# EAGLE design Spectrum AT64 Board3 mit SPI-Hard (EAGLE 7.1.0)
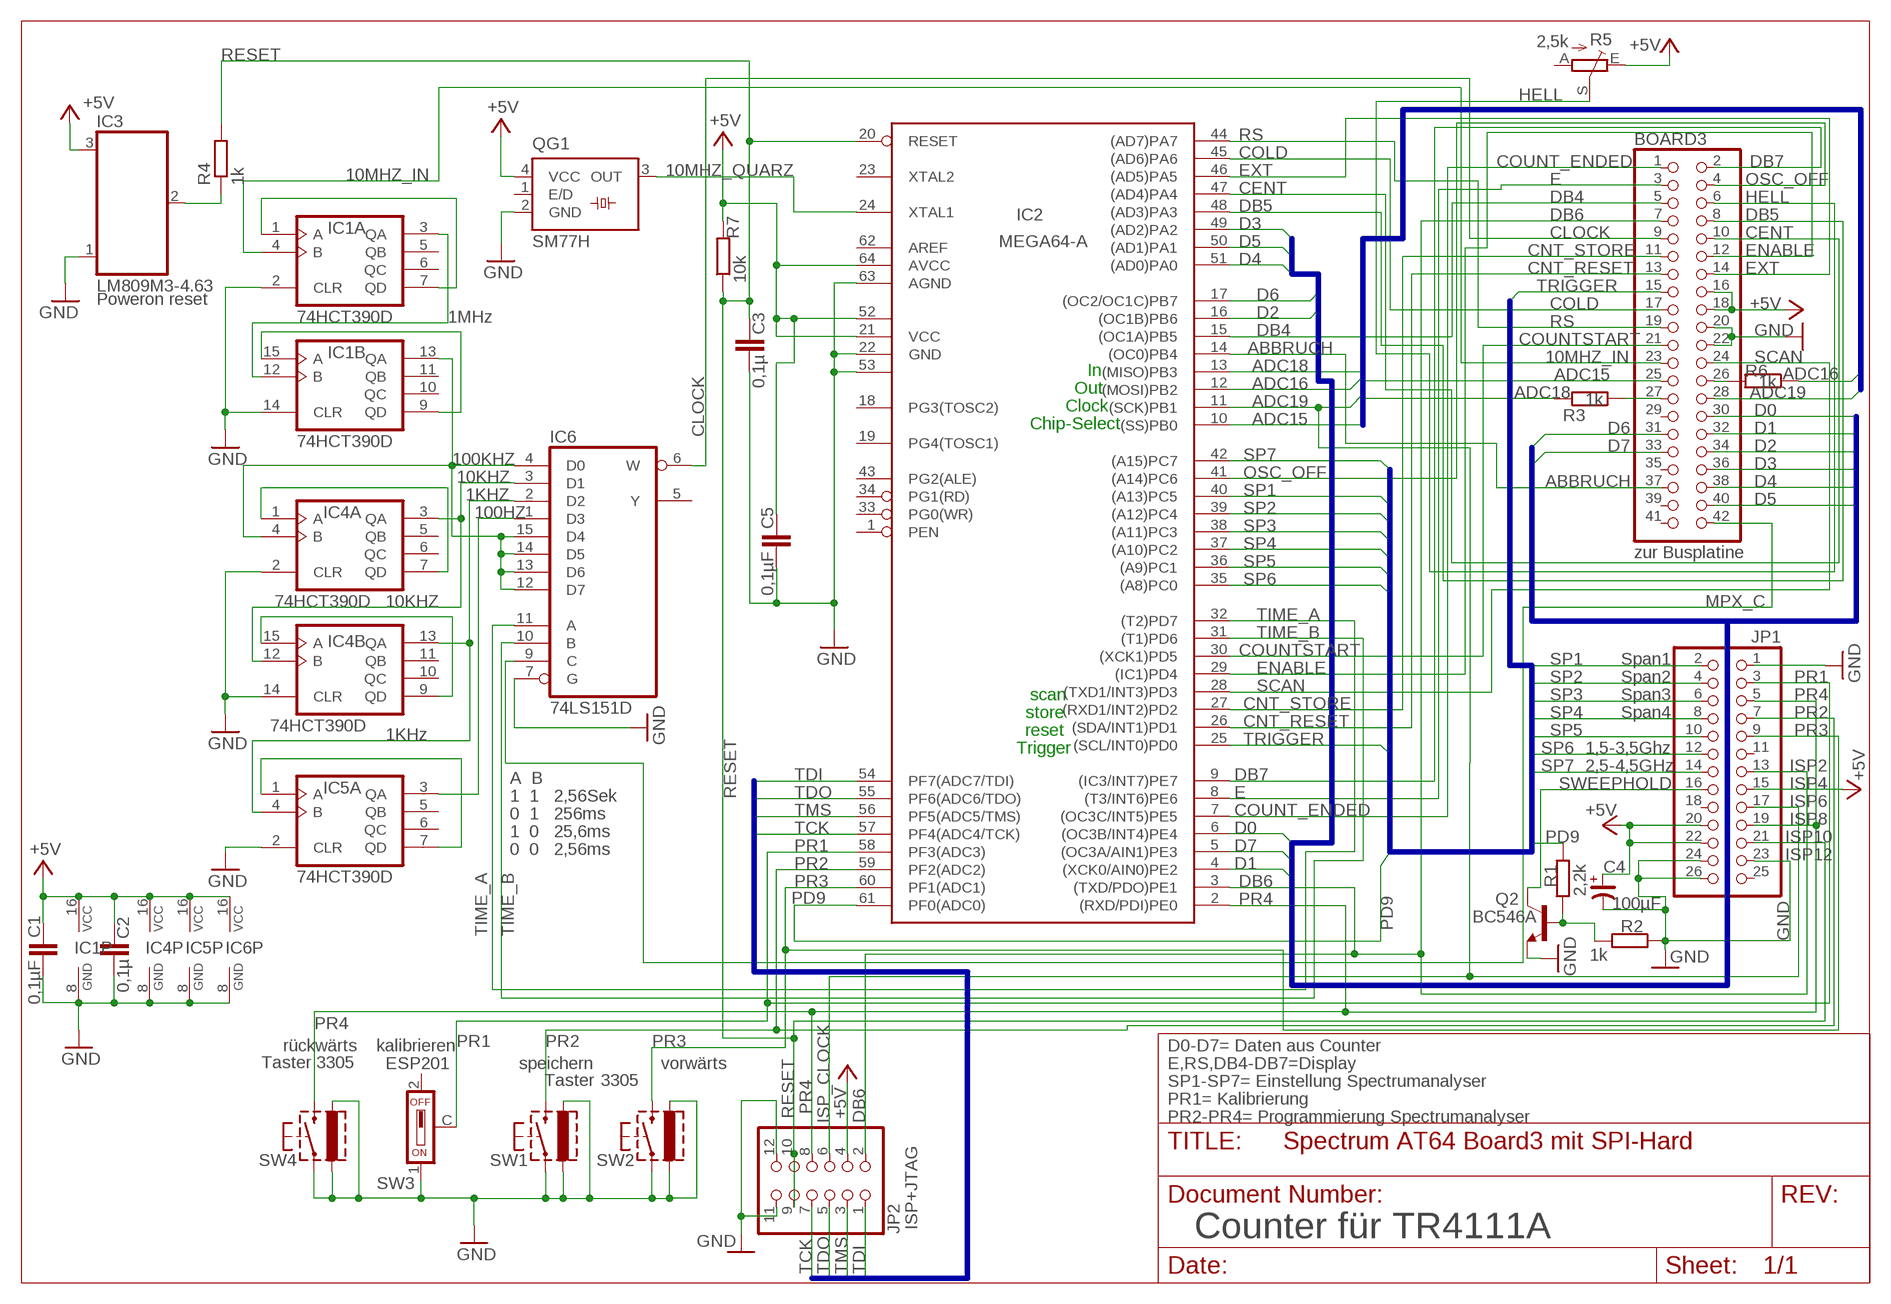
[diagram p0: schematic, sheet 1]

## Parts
BOARD3  zur Busplatine  PINHD-2X21_2.54-90°  [2X21/90]
C1  0,1µF  C-EUC0805  [C0805]
C2  0,1µ  C-EU025-025X050  [C025-025X050]
C3  0,1µ  C-EUC0805K  [C0805K]
C4  100µF  CP_SV-D  [CSV-D]
C5  0,1µF  C-EUC0805  [C0805]
IC1  74HCT390D  [SO16]
IC2  MEGA64-A  [TQFP64]
IC3  LM809M3-4.63  [SOT23]
IC4  74HCT390D  [SO16]
IC5  74HCT390D  [SO16]
IC6  74LS151D  74S151D  [SO16]
JP1  PINHD-2X13_2.54-90°  [2X13/90]
JP2  ISP+JTAG  PINHD-2X06_2.54-90°  [2X06/90]
Q2  BC546A  [TO92-EBC]
QG1  SM77H  [SM77H]
R1  2,2k  R-EU_R0805  [R0805]
R2  1k  R-EU_R0805  [R0805]
R3  1k  R-EU_R0805  [R0805]
R4  1k  R-EU_R0805  [R0805]
R5  2,5k  TRIM_EU-CA6H  [CA6H]
R6  1k  R-EU_R0805  [R0805]
R7  10k  WIDERSTAND_10  [207.10]
SW1  Taster  SW-PUSH-90  [SW-PUSH-90]
SW2  3305  SW-PUSH-90  [SW-PUSH-90]
SW3  ESP201  [ESP201]
SW4  Taster 3305  SW-PUSH-90  [SW-PUSH-90]

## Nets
1KHZ: IC4.13(B:QA) IC5.4(A:B) IC6.2(D2)
1MHZ: IC1.3(A:QA) IC1.12(B:B)
10KHZ: IC4.3(A:QA) IC4.12(B:B) IC6.3(D1)
10MHZ_IN: BOARD3.23 IC1.4(A:B)
10MHZ_QUARZ: IC2.24(XTAL1) QG1.3(OUT)
100HZ: IC5.3(A:QA) IC6.1(D3)
100KHZ: IC1.13(B:QA) IC4.4(A:B) IC6.4(D0) IC6.12(D7) IC6.13(D6) IC6.14(D5) IC6.15(D4)
+5V: BOARD3.16 BOARD3.18 C1.2 C2.1 C4.+ C5.2 IC1.16(P:VCC) IC2.21(VCC) IC2.52(VCC1) IC2.64(AVCC) IC3.3(VCC) IC4.16(P:VCC) IC5.16(P:VCC) IC6.16(VCC) JP1.15 JP1.20 JP1.22 JP2.4 QG1.4(VCC) R5.E R7.2
ABBRUCH: BOARD3.37 IC2.14((OC0)PB4)
ADC15: BOARD3.25 IC2.10((SS)PB0)
ADC16: IC2.12((MOSI)PB2) R6.1
ADC18: IC2.13((MISO)PB3) R3.2
ADC19: BOARD3.28 IC2.11((SCK)PB1) JP1.17 JP2.6
CENT: BOARD3.10 IC2.47((AD4)PA4)
CLOCK: BOARD3.9 IC6.6(W)
CNT_RESET: BOARD3.13 IC2.26((SDA/INT1)PD1)
CNT_STORE: BOARD3.11 IC2.27((RXD1/INT2)PD2)
COLD: BOARD3.17 IC2.45((AD6)PA6)
COUNT_ENDED: BOARD3.1 IC2.7((OC3C/INT5)PE5)
COUNTSTART: BOARD3.21 IC2.30((XCK1)PD5)
D0: BOARD3.30 IC2.6((OC3B/INT4)PE4)
D1: BOARD3.32 IC2.4((XCK0/AIN0)PE2)
D2: BOARD3.34 IC2.16((OC1B)PB6)
D3: BOARD3.36 IC2.49((AD2)PA2)
D4: BOARD3.38 IC2.51((AD0)PA0)
D5: BOARD3.40 IC2.50((AD1)PA1)
D6: BOARD3.31 IC2.17((OC2/OC1C)PB7)
D7: BOARD3.33 IC2.5((OC3A/AIN1)PE3)
DB4: BOARD3.5 IC2.15((OC1A)PB5)
DB5: BOARD3.8 IC2.48((AD3)PA3)
DB6: BOARD3.7 IC2.3((TXD/PDO)PE1) JP1.13 JP2.2
DB7: BOARD3.2 IC2.9((IC3/INT7)PE7)
E: BOARD3.3 IC2.8((T3/INT6)PE6)
ENABLE: BOARD3.12 IC2.29((IC1)PD4)
EXT: BOARD3.14 IC2.46((AD5)PA5)
GND: BOARD3.20 BOARD3.22 C1.1 C2.2 C3.2 C4.- C5.1 IC1.2(A:CLR) IC1.8(P:GND) IC1.14(B:CLR) IC2.22(GND) IC2.53(GND1) IC2.63(AGND) IC3.1(GND) IC4.2(A:CLR) IC4.8(P:GND) IC4.14(B:CLR) IC5.2(A:CLR) IC5.8(P:GND) IC6.7(G) IC6.8(GND) JP1.1 JP1.23 JP1.24 JP1.26 JP2.11 JP2.12 Q2.E QG1.2(GND) R2.1 SW1.1 SW1.3(G1) SW1.4(G2) SW2.1 SW2.3(G1) SW2.4(G2) SW3.1 SW4.1 SW4.3(G1) SW4.4(G2)
HELL: BOARD3.6 R5.S
MPX_C: BOARD3.42 IC6.9(C)
N$2: IC3.2(/RESET) R4.1
N$4: IC1.1(A:A) IC1.7(A:QD)
N$5: BOARD3.27 R3.1
N$6: Q2.B R1.1 R2.2
N$7: BOARD3.26 R6.2
N$11: IC1.9(B:QD) IC1.15(B:A)
N$15: IC5.1(A:A) IC5.7(A:QD)
N$17: IC4.1(A:A) IC4.7(A:QD)
N$18: IC4.9(B:QD) IC4.15(B:A)
OSC_OFF: BOARD3.4 IC2.41((A14)PC6)
PD9: IC2.61(PF0(ADC0)) R1.2
PR1: IC2.58(PF3(ADC3)) JP1.3 SW3.C
PR2: IC2.59(PF2(ADC2)) JP1.7 SW1.2(S1)
PR3: IC2.60(PF1(ADC1)) JP1.9 SW2.2(S1)
PR4: IC2.2((RXD/PDI)PE0) JP1.5 JP1.19 JP2.8 SW4.2(S1)
RESET: C3.1 IC2.20(RESET) JP1.21 JP2.9 JP2.10 R4.2 R7.1
RS: BOARD3.19 IC2.44((AD7)PA7)
SCAN: BOARD3.24 IC2.28((TXD1/INT3)PD3)
SP1: IC2.40((A13)PC5) JP1.2
SP2: IC2.39((A12)PC4) JP1.4
SP3: IC2.38((A11)PC3) JP1.6
SP4: IC2.37((A10)PC2) JP1.8
SP5: IC2.36((A9)PC1) JP1.10
SP6: IC2.35((A8)PC0) JP1.12
SP7: IC2.42((A15)PC7) JP1.14
SWEEPHOLD: JP1.16 Q2.C
TCK: IC2.57(PF4(ADC4/TCK)) JP2.7
TDI: IC2.54(PF7(ADC7/TDI)) JP2.1
TDO: IC2.55(PF6(ADC6/TDO)) JP2.5
TIME_A: IC2.32((T2)PD7) IC6.11(A)
TIME_B: IC2.31((T1)PD6) IC6.10(B)
TMS: IC2.56(PF5(ADC5/TMS)) JP2.3
TRIGGER: BOARD3.15 IC2.25((SCL/INT0)PD0)
Unconnected: BOARD3.29 BOARD3.35 BOARD3.39 BOARD3.41 IC1.5(A:QB) IC1.6(A:QC) IC1.10(B:QC) IC1.11(B:QB) IC2.1(PEN) IC2.18(PG3(TOSC2)) IC2.19(PG4(TOSC1)) IC2.23(XTAL2) IC2.33(PG0(WR)) IC2.34(PG1(RD)) IC2.43(PG2(ALE)) IC2.62(AREF) IC4.5(A:QB) IC4.6(A:QC) IC4.10(B:QC) IC4.11(B:QB) IC5.5(A:QB) IC5.6(A:QC) IC5.9(B:QD) IC5.10(B:QC) IC5.11(B:QB) IC5.12(B:B) IC5.13(B:QA) IC5.14(B:CLR) IC5.15(B:A) IC6.5(Y) JP1.11 JP1.18 JP1.25 QG1.1(E/D) R5.A SW3.2

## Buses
ADC[15..19]
D[0..7]
SP[1..10],TRIGGER,PD9
TDI,TDO,TMS,TCK,RESET

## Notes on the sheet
- Poweron reset
- 1MHz
- In
- Out
- Clock
- Chip-Select
- 10KHZ
- Span1
- Span2
- scan | Span3
- store | Span4
- 1KHz | reset
- Trigger | 1,5-3,5Ghz
- A  B | 2,5-4,5GHz | ISP2
- 1  1   2,56Sek | ISP4
- 0  1   256ms | ISP6
- 1  0   25,6ms | ISP8
- 0  0   2,56ms | ISP10
- ISP12
- rückwärts | kalibrieren | D0-D7= Daten aus Counter
- speichern | vorwärts | E,RS,DB4-DB7=Display
- SP1-SP7= Einstellung Spectrumanalyser
- PR1= Kalibrierung
- ISP_CLOCK | PR2-PR4= Programmierung Spectrumanalyser
- Counter für TR4111A

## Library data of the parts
BOARD3 = pinhead-2:PINHD-2X21: PIN HEADER
C1-C3 C5 = rcl:C-EU: CAPACITOR, European symbol
C4 = rc-master-smd:CP_: POLARIZED CAP
IC1 IC4 IC5 = 74xx-eu:74*390: Dual 4-bit decade and binary COUNTER
IC2 = atmel:MEGA64: MICROCONTROLLER 64 Kbytes FLASH 4 Kbytes SRAM 2 Kbytes EEPROM DUAL USART 8-channel 10 bit ADC Source: avr.lbr
IC3 = 1Eigene:LM809M3-4.63
IC6 = 74xx-eu:74*151: Data SELECTOR/MULTIPLEXER
JP1 = pinhead-2:PINHD-2X13: PIN HEADER
JP2 = pinhead-2:PINHD-2X06: PIN HEADER
Q2 = transistor-npn:BC546*: NPN Transistor
QG1 = crystal:SM77H: 3.3V CMOS Clock Oscillator Source: www.pletronics.com .. sm77h%203.3v.pdf
R1-R4 R6 = rcl:R-EU_: RESISTOR, European symbol
R5 = pot:TRIM_EU-: POTENTIOMETER
R7 = 1Eigene:WIDERSTAND_10
SW1 SW2 SW4 = 1Eigene:SW-PUSH-90
SW3 = 1Eigene:ESP201

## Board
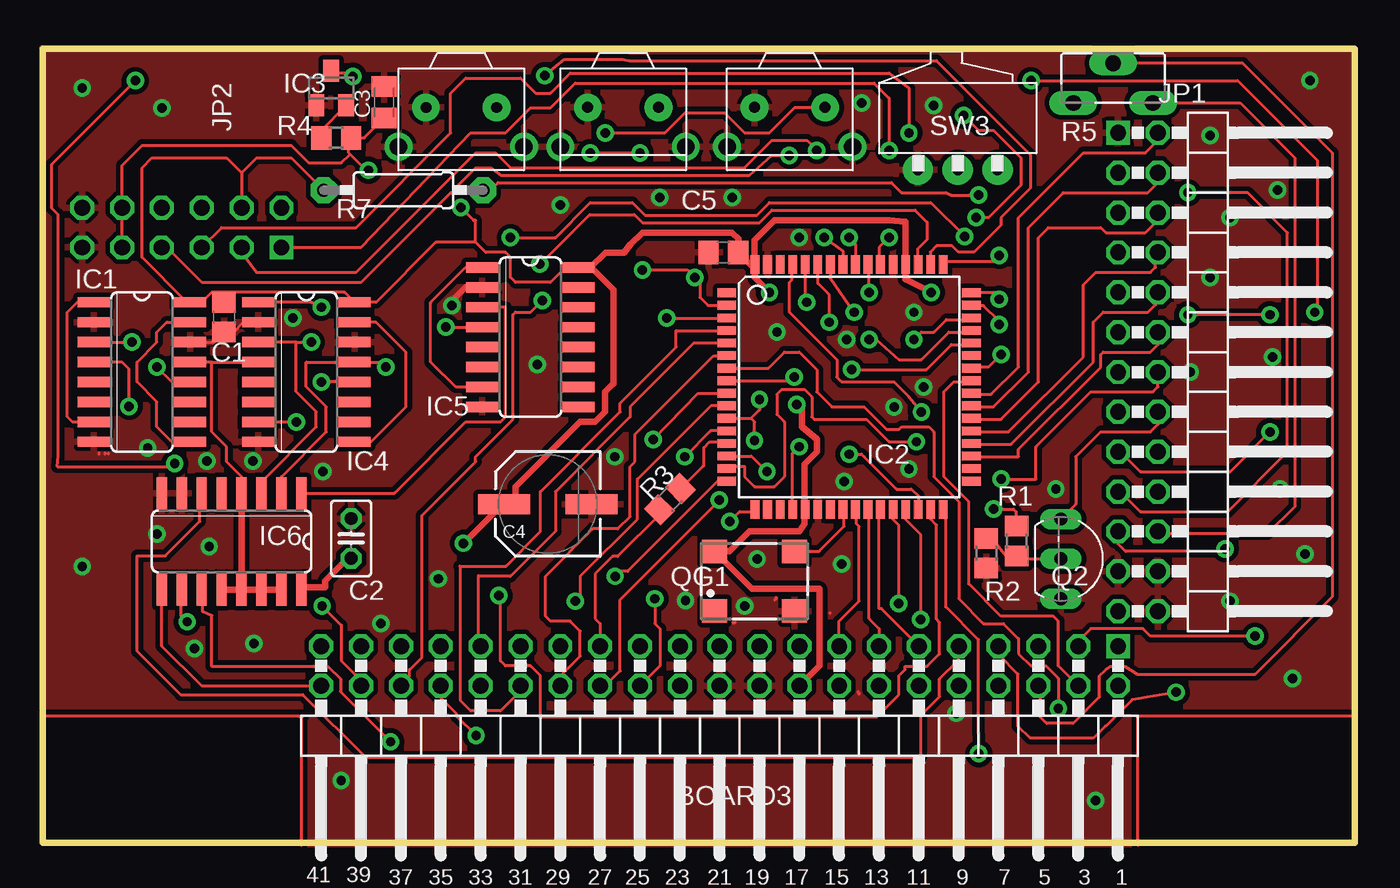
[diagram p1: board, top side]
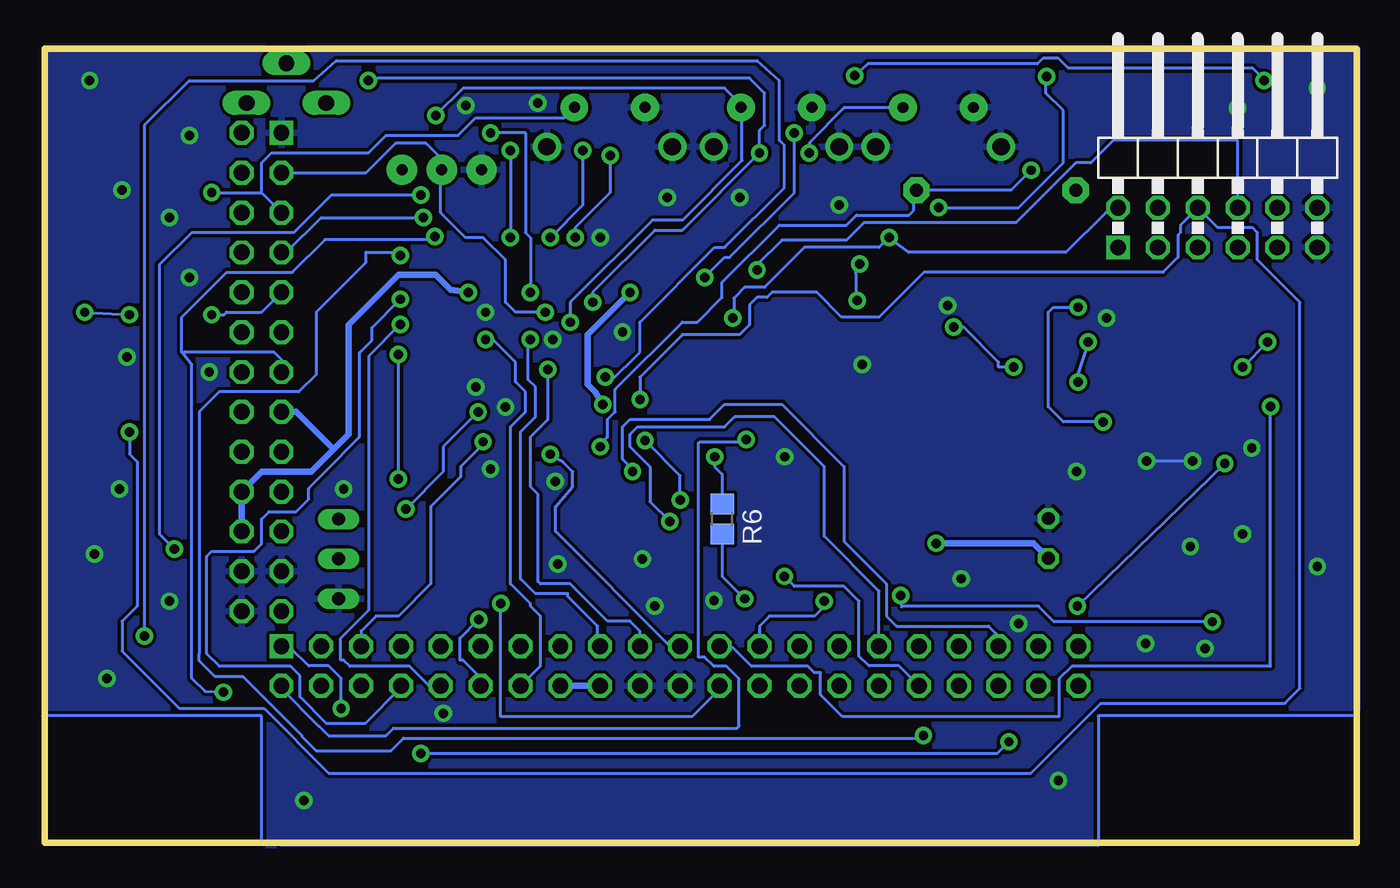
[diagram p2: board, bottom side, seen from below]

Size 83.63 x 50.58 mm. Coordinates in mm from the lower left corner, seen from the top.
Outline: 0,0 83.63,0 83.63,50.58 0,50.58 0,0
Copper layers (1*16): Top 0.035mm / dielectric 1.5mm / Bottom 0.035mm
Design rules "default *": minimum track width 0.2mm, minimum drill 0.6mm, track to track 0.2mm, track to pad 0.2mm, pad to pad 0.2mm, via to via 0.2mm, smd to smd 0.2mm, copper to edge 0mil, drill to drill 0.4mm, minimum pad ring 10mil, minimum via ring 10mil, stop-mask expansion 4mil, vias tented up to drill 0mil, thermal gap 10mil

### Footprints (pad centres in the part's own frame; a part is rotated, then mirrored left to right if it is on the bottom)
2X21/90 = drill 1.016 square: 1 -24.13,-6.35 | drill 1.016 octagon: 2 -24.13,-3.81; 3 -21.59,-6.35; 4 -21.59,-3.81; 5 -19.05,-6.35; 6 -19.05,-3.81; 7 -16.51,-6.35; 8 -16.51,-3.81; 9 -13.97,-6.35; 10 -13.97,-3.81; 11 -11.43,-6.35; 12 -11.43,-3.81; 13 -8.89,-6.35; 14 -8.89,-3.81; 15 -6.35,-6.35; 16 -6.35,-3.81; 17 -3.81,-6.35; 18 -3.81,-3.81; 19 -1.27,-6.35; 20 -1.27,-3.81; 21 1.27,-6.35; 22 1.27,-3.81; 23 3.81,-6.35; 24 3.81,-3.81; 25 6.35,-6.35; 26 6.35,-3.81; 27 8.89,-6.35; 28 8.89,-3.81; 29 11.43,-6.35; 30 11.43,-3.81; 31 13.97,-6.35; 32 13.97,-3.81; 33 16.51,-6.35; 34 16.51,-3.81; 35 19.05,-6.35; 36 19.05,-3.81; 37 21.59,-6.35; 38 21.59,-3.81; 39 24.13,-6.35; 40 24.13,-3.81; 41 26.67,-6.35; 42 26.67,-3.81
C0805 = smd 1.3 x 1.5: 1 -0.95,0; 2 0.95,0
C025-025X050 = drill 0.813 octagon: 1 -1.27,0; 2 1.27,0
C0805K = smd 1.3 x 1.6: 1 -1,0; 2 1,0
CSV-D = smd 3.302 x 1.27: + -2.794,0; - 2.794,0
SO16 = smd 0.66 x 2.032: 1 -4.445,-3.073; 2 -3.175,-3.073; 3 -1.905,-3.073; 4 -0.635,-3.073; 5 0.635,-3.073; 6 1.905,-3.073; 7 3.175,-3.073; 8 4.445,-3.073; 9 4.445,3.073; 10 3.175,3.073; 11 1.905,3.073; 12 0.635,3.073; 13 -0.635,3.073; 14 -1.905,3.073; 15 -3.175,3.073; 16 -4.445,3.073
TQFP64 = smd 1.194 x 0.559: 1 -7.8,6; 2 -7.8,5.2; 3 -7.8,4.4; 4 -7.8,3.6; 5 -7.8,2.8; 6 -7.8,2; 7 -7.8,1.2; 8 -7.8,0.4; 9 -7.8,-0.4; 10 -7.8,-1.2; 11 -7.8,-2; 12 -7.8,-2.8; 13 -7.8,-3.6; 14 -7.8,-4.4; 15 -7.8,-5.2; 16 -7.8,-6; 33 7.8,-6; 34 7.8,-5.2; 35 7.8,-4.4; 36 7.8,-3.6; 37 7.8,-2.8; 38 7.8,-2; 39 7.8,-1.2; 40 7.8,-0.4; 41 7.8,0.4; 42 7.8,1.2; 43 7.8,2; 44 7.8,2.8; 45 7.8,3.6; 46 7.8,4.4; 47 7.8,5.2; 48 7.8,6 | smd 0.559 x 1.194: 17 -6,-7.8; 18 -5.2,-7.8; 19 -4.4,-7.8; 20 -3.6,-7.8; 21 -2.8,-7.8; 22 -2,-7.8; 23 -1.2,-7.8; 24 -0.4,-7.8; 25 0.4,-7.8; 26 1.2,-7.8; 27 2,-7.8; 28 2.8,-7.8; 29 3.6,-7.8; 30 4.4,-7.8; 31 5.2,-7.8; 32 6,-7.8; 49 6,7.8; 50 5.2,7.8; 51 4.4,7.8; 52 3.6,7.8; 53 2.8,7.8; 54 2,7.8; 55 1.2,7.8; 56 0.4,7.8; 57 -0.4,7.8; 58 -1.2,7.8; 59 -2,7.8; 60 -2.8,7.8; 61 -3.6,7.8; 62 -4.4,7.8; 63 -5.2,7.8; 64 -6,7.8
SOT23 = smd 1 x 1.4: 1 -0.95,-1.1; 2 0.95,-1.1; 3 0,1.1
2X13/90 = drill 1.016 square: 1 -15.24,-6.35 | drill 1.016 octagon: 2 -15.24,-3.81; 3 -12.7,-6.35; 4 -12.7,-3.81; 5 -10.16,-6.35; 6 -10.16,-3.81; 7 -7.62,-6.35; 8 -7.62,-3.81; 9 -5.08,-6.35; 10 -5.08,-3.81; 11 -2.54,-6.35; 12 -2.54,-3.81; 13 0,-6.35; 14 0,-3.81; 15 2.54,-6.35; 16 2.54,-3.81; 17 5.08,-6.35; 18 5.08,-3.81; 19 7.62,-6.35; 20 7.62,-3.81; 21 10.16,-6.35; 22 10.16,-3.81; 23 12.7,-6.35; 24 12.7,-3.81; 25 15.24,-6.35; 26 15.24,-3.81
2X06/90 = drill 1.016 square: 1 -6.35,-6.35 | drill 1.016 octagon: 2 -6.35,-3.81; 3 -3.81,-6.35; 4 -3.81,-3.81; 5 -1.27,-6.35; 6 -1.27,-3.81; 7 1.27,-6.35; 8 1.27,-3.81; 9 3.81,-6.35; 10 3.81,-3.81; 11 6.35,-6.35; 12 6.35,-3.81
TO92-EBC = drill 0.813 long: B 0,-1.27; C -2.54,-1.27; E 2.54,-1.27
SM77H = smd 1.6 x 1.5: 1 -2.55,-1.9; 2 2.55,-1.9; 3 2.55,1.9; 4 -2.55,1.9
R0805 = smd 1.3 x 1.5: 1 -0.95,0; 2 0.95,0
CA6H = drill 1.016 long: A -2.54,0; E 2.54,0; S 0,2.54
207.10 = drill 0.813 pad 1.676 octagon: 1 -5.08,0; 2 5.08,0
SW-PUSH-90 = drill 0.7 pad 1.778: 1 1.75,4; 2 6.25,4 | drill 1.1 pad 1.778: 3 0,1.5; 4 8,1.5
ESP201 = drill 0.7 pad 1.93: 1 -2.54,-2.54; 2 2.54,-2.54; C 0,-2.54

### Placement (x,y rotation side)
BOARD3  44.42,6.17 180 top
C1  11.56,33.48 90 top
C2  19.66,19.38 90 top
C3  21.77,47.18 90 top
C4  32.2,21.57 0 top
C5  43.39,37.6 0 top
IC1  6.32,29.98 270 top
IC2  51.41,29.03 0 top
IC3  18.39,48.08 0 top
IC4  16.8,29.98 270 top
IC5  31.09,32.21 270 top
IC6  12.04,19.19 180 top
JP1  74.9,29.98 270 top
JP2  8.86,44.27 0 bottom
Q2  66.17,18.08 270 top
QG1  45.38,16.65 0 top
R1  62.09,19.21 90 top
R2  60.15,18.44 90 top
R3  39.98,21.89 45 top
R4  18.71,44.91 0 top
R5  68.24,47.13 0 top
R6  40.46,20.62 270 bottom
R7  22.99,41.57 180 top
SW1  32.99,42.84 0 top
SW2  22.68,42.84 0 top
SW3  58.33,45.42 0 top
SW4  43.63,42.84 0 top

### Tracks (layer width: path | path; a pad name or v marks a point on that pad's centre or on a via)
1KHZ  (via drill 0.6 pad 0.7)
  Top 0.2: IC6.2 15.21,23.32 18.07,26.17 18.07,27.76 16.8,29.03 16.8,30.62 IC4.13 21.56,30.62 v21.88,30.3 | v25.69,32.84 IC5.4
  Bottom 0.2: v21.88,30.3 22.83,30.3 22.83,30.62 25.06,32.84 v25.69,32.84
1MHZ  (via drill 0.6 pad 0.7)
  Top 0.2: IC1.12 9.5,29.4 8.18,29.4 v7.28,30.3 | IC1.3 v5.69,31.89
  Bottom 0.2: v5.69,31.89 v7.28,30.3
10KHZ  (via drill 0.6 pad 0.7)
  Top 0.2: IC4.12 19.95,29.4 17.8,29.4 v17.75,29.35 | IC6.3 13.94,23 17.44,26.49 17.44,27.44 16.17,28.71 16.17,31.89 | 16.17,31.89 IC4.3 | 16.17,31.89 v17.12,31.89
  Bottom 0.2: v17.75,29.35 17.75,29.99 v17.12,31.89
10MHZ_IN  (via drill 0.6 pad 0.7)
  Top 0.2: v5.5,27.8 5.5,30.17 5.05,30.62 IC1.4
  Bottom 0.2: v5.5,27.8 5.5,11.22 18.17,11.22 18.97,10.42 18.97,8.02 32.77,8.02 34.17,9.42 34.17,10.82 34.57,10.82 34.97,11.22 38.57,11.22 39.77,12.42 40.57,12.42 BOARD3.23
10MHZ_QUARZ
  Top 0.2: QG1.3 49.5,18.55 51.09,20.14 51.09,21.15 IC2.24
100HZ
  Top 0.2: IC6.1 16.61,22.27 22.42,22.27 26.96,26.81 29.18,26.81 29.5,27.13 29.5,34.11 IC5.3
100KHZ
  Top 0.2: IC6.4 12.67,23.32 11.72,24.27 11.72,25.22 10.77,26.17 10.77,30.62 | 10.77,30.62 IC1.13 | 10.77,30.62 IC4.4
  Top 0.406: IC6.15 IC6.14 IC6.13 | IC6.12 IC6.13 | IC6.13 IC6.4
+5V  (via drill 0.6 pad 0.7)
  Top 0.2: 45.11,36.83 IC2.64 45.38,36.86 | IC2.21 48.55,21.17 | 48.55,21.29 IC2.21 | IC2.21 48.55,21.13 | 49.5,11.41 49.5,11.25 | IC6.16 16.61,16.27 | 19.61,18.27 C2.1 | 30.97,21.62 30.14,21.62 29.57,21.62 C4.+ 29.37,21.62 | IC4.16 19.75,34.6 | v19.77,48.82 19.77,49.02 18.57,49.02 IC3.3 | IC4.16 19.95,34.6 | 34.97,36.62 34.9,36.62 34.17,36.62 IC5.16 33.97,36.82 33.48,36.82 32.36,35.7 30.14,35.7 29.82,36.02 29.82,37.29 29.5,37.6 28.23,37.6 27.6,38.24 | 36.36,29.22 36.37,29.22 | R7.2 15.85,43.64 13.63,43.64 12.67,42.68 | 12.67,42.68 JP2.4 | 11.56,35.06 19.24,35.06 IC4.16 | 11.56,35.06 10.77,35.06 10.13,34.43 IC1.16 9.18,34.43 6.32,37.29 6.32,43 6.96,43.64 11.72,43.64 12.67,42.68 | 27.6,38.24 27.6,39.64 27.46,39.64 v26.64,40.46 | 27.6,38.24 25.06,38.24 21.25,34.43 IC4.16 | R5.E 76.33,47.13 79.83,43.64 79.83,21.41 78.08,19.67 71.25,19.67 JP1.22 | C1.2 11.56,35.06
  Top 0.406: 45.11,36.83 C5.2 44.34,38.48 43.95,38.88 38.23,38.88 37.48,38.12 37.06,37.59 35.86,37.59 34.9,36.62 | IC2.64 45.41,35.99 v46.33,35.06 | 45.38,36.86 45.38,38.4 46.65,39.67 53.95,39.67 55.01,39.56 IC2.52 55.01,35.91 v56.65,35.06 | 49.5,11.41 49.5,14.27 49.5,16.17 45.2,16.17 QG1.4 43.79,18.56 45.06,19.83 48.23,19.83 48.55,20.3 48.55,21.13 | 49.5,11.25 BOARD3.18 | 16.61,16.27 18.01,16.27 18.01,16.67 19.61,18.27 | v26.82,19.07 29.37,21.62 | 36.37,29.22 36.37,35.22 34.97,36.62 | 36.36,29.22 35.85,28.71 35.85,27.44 35.22,26.81 34.26,26.81 30.14,22.68 30.14,21.62 | 48.55,21.29 48.55,24.11 49.35,24.9 49.35,25.7 48.39,26.49 48.39,27.76 v48.08,27.92
  Bottom 0.2: v26.64,40.46 21.56,40.46 18.71,43.32 18.71,46.65 19.82,47.77 19.82,48.78 v19.77,48.82
  Bottom 0.406: v56.65,35.06 57.76,35.22 58.71,36.18 61.09,36.18 64.27,33 64.27,26.02 65.22,25.06 | BOARD3.18 BOARD3.16 | v26.82,19.07 20.61,19.07 19.81,18.27 C2.1 | JP1.22 JP1.20 69.82,23.63 66.65,23.63 65.22,25.06 | JP1.15 67.6,27.44 65.22,25.06 | v46.33,35.06 49.03,32.37 49.03,29.19 48.55,28.72 v48.08,27.92
ABBRUCH  (via drill 0.6)
  Top 0.2: IC2.14 45.17,24.63 v46.17,23.63
  Bottom 0.2: v46.17,23.63 46.17,23.79 46.81,24.43 46.81,26.49 46.33,26.97 41.25,26.97 40.3,27.92 36.65,27.92 32.68,23.95 32.68,19.19 29.98,16.49 29.98,14.43 29.34,13.79 23.47,13.79 22.99,13.32 22.99,12.68 BOARD3.37
ADC15  (via drill 0.6 pad 0.7)
  Top 0.2: v33.95,15.38 34.26,15.7 34.26,16.97 37.92,20.62 37.92,23.16 42.59,27.83 IC2.10
  Bottom 0.2: v33.95,15.38 33.95,15.06 34.58,14.43 37.44,14.43 38.07,13.79 BOARD3.25
ADC16  (via drill 0.6 pad 0.7)
  Top 0.2: IC2.12 42.58,26.23 v40.93,24.59
  Bottom 0.2: v40.93,24.59 40.93,23.95 40.46,23.48 R6.1
ADC18
  Top 0.2: IC2.13 43.5,25.54 42.52,25.54 42.14,25.16 42.14,23.99 42.08,23.99 R3.2
ADC19  (via drill 0.6, 0.6 pad 0.7)
  Top 0.2: v45.37,25.62 45.37,26.81 45.15,27.03 | v43.14,21.82 36.8,15.49 36.8,10.94 35.85,9.98 BOARD3.28 | IC2.11 45.15,27.03 | JP1.17 68.71,24.9 69.98,23.63 75.7,23.63 v78.24,26.17 | v45.69,28.24 45.69,27.58 45.15,27.03
  Bottom 0.2: v43.14,21.82 43.14,23.39 v45.37,25.62 | v78.24,26.17 78.24,24.75 77.76,24.27 77.76,15.06 78.71,14.11 78.71,12.21 75.06,8.55 69.67,8.55 65.54,4.43 20.77,4.43 16.33,8.87 4.58,8.87 3.63,9.82 3.63,34.43 6.32,37.13 6.32,38.88 6.64,39.19 8.86,39.19 JP2.6 11.25,39.35 11.25,38.88 11.4,38.72 11.4,37.29 12.36,36.34 27.6,36.34 30.45,33.48 32.84,33.48 34.42,35.06 37.28,35.06 37.6,34.75 38.23,34.75 38.71,34.27 38.71,33 39.34,32.37 43,32.37 45.69,29.67 v45.69,28.24
CENT  (via drill 0.6 pad 0.7)
  Top 0.2: v60.97,33.02 60.97,33.22 59.97,34.22 59.37,34.22 IC2.47
  Bottom 0.2: v60.97,33.02 62.97,31.02 62.97,14.82 64.77,13.02 64.77,11.62 64.57,11.62 64.17,11.22 60.37,11.22 59.17,10.02 58.57,10.02 BOARD3.10
CLOCK
  Top 0.2: IC6.6 10.01,22.07 10.01,20.47 7.81,18.27 6.01,18.27 6.01,14.87 6.01,12.21 8.79,9.42 16.57,9.42 20.57,5.42 55.97,5.42 55.97,8.11 57.17,9.3 57.17,10.42 58.37,11.62 58.37,12.42 BOARD3.9
CNT_RESET
  Top 0.2: IC2.26 52.68,21.16 52.68,14.27 53.31,13.63 BOARD3.13
CNT_STORE
  Top 0.2: IC2.27 53.31,21.14 53.31,14.9 53.47,14.9 BOARD3.11
COLD  (via drill 0.6 pad 0.7)
  Top 0.2: v52.68,32.05 53.16,32.05 54.58,30.78 56.01,30.78 57.76,32.53 59.1,32.53 IC2.45
  Bottom 0.2: v52.68,32.05 52.84,31.89 52.84,29.51 52.36,29.03 52.36,27.13 53.31,26.17 53.31,16.81 52.36,15.86 50.3,15.86 50.3,15.7 48.39,13.79 48.39,12.68 BOARD3.17
COUNT_ENDED  (via drill 0.6)
  Top 0.2: IC2.7 46.26,30.23 47.28,31.26 48.23,31.26 49.35,30.14 49.35,28.71 50.3,27.76 52.36,27.76 53.79,26.33 54.58,26.33 54.74,26.49 56.49,26.49 56.81,26.17 56.81,23.32 58.39,21.73 58.39,15.54 59.98,13.95 61.25,13.95 62.2,13 62.2,12.05 63,11.25 63.95,11.25 64.74,10.46 v64.74,8.55
  Bottom 0.2: v64.74,8.55 64.74,10.46 65.54,11.25 66.81,11.25 67.92,12.36 68.4,12.36 BOARD3.1
COUNTSTART  (via drill 0.6 pad 0.7)
  Top 0.2: IC2.30 55.81,22.09 55.38,22.52 54.43,22.52 52.36,24.59 | 52.36,24.59 | 52.36,24.59 52.2,24.75 v51.41,24.75
  Bottom 0.2: BOARD3.21 43.79,12.52 51.09,19.83 51.09,21.41 49.98,22.68 49.98,23.63 50.62,24.27 51.25,24.59 v51.41,24.75
D0
  Top 0.2: IC2.6 43.57,31.02 42.77,31.02 37.76,26.01 37.76,24.27 37.44,23.95 37.44,20.78 36.65,19.98 35.06,19.98 32.04,16.97 32.04,14.43 32.36,14.11 33.63,14.11 34.26,13.47 34.26,11.89 32.99,10.62 BOARD3.30
D1
  Top 0.2: IC2.4 43.57,32.62 40.37,32.62 40.37,31.57 36.8,28 36.8,27.44 31.72,22.37 31.72,19.83 29.52,17.62 26.57,17.62 26.64,17.55 26.64,9.03 27.28,8.39 29.18,8.39 30.45,9.66 BOARD3.32
D2  (via drill 0.6 pad 0.7)
  Top 0.2: IC2.16 43.58,23 43,23 37.28,17.28 36.8,17.28 v36.49,16.97
  Bottom 0.2: v36.49,16.97 35.85,16.33 32.68,16.33 31.72,15.38 31.72,11.89 31.09,11.25 29.18,11.25 BOARD3.34
D3  (via drill 0.6 pad 0.7)
  Top 0.2: v60.97,37.42 60.97,37.02 57.57,37.02 IC2.49 | v27.62,6.82 26.42,8.02 26.37,8.02 26.37,8.22 25.37,9.22 BOARD3.36
  Bottom 0.2: v60.97,37.42 61.17,37.62 63.17,37.62 63.17,36.95 66.33,33.79 66.33,29.83 67.44,28.71 72.52,28.71 73.79,27.44 73.79,26.24 73.77,26.22 73.77,12.06 73.79,12.04 73.79,11.57 72.79,10.57 71,10.57 67.26,6.82 67.26,6.78 66.33,5.85 61.57,5.85 60.78,6.65 27.8,6.65 v27.62,6.82
D4  (via drill 0.6 pad 0.7)
  Top 0.2: IC2.51 55.77,37.02 55.77,37.82 56.37,38.42 56.37,39.54 55.61,40.3 46.49,40.3 45.69,39.51 38.23,39.51 37.72,40.02 34.86,40.02 v31.69,36.86 | BOARD3.38 22.97,10.02 22.97,10.22 23.37,10.62 23.37,11.02 24.17,11.82 24.17,20.85 27.6,24.27 27.6,24.59 29.98,26.97 29.98,33.64 30.14,33.79 31.1,33.79 v31.86,34.55
  Bottom 0.2: v31.69,36.86 31.93,36.78 v31.86,34.55
D5  (via drill 0.6 pad 0.7)
  Top 0.2: v32,48.87 33.27,49.91 36.97,49.91 37.37,49.82 56.97,49.82 62.97,43.82 62.97,41.71 61.09,39.82 61.09,39.81 61.09,39.35 59.36,37.62 58.37,37.62 57.97,38.02 56.97,38.02 56.57,37.62 56.57,37.02 IC2.50 | v5.9,48.55 0.57,43.22 0.57,40.42 0.97,40.02 0.97,24.63 0.93,23.95 8.29,23.95 v8.41,24.15 | v17.81,15.07 19.02,13.86 19.02,11.57 20.29,10.3 BOARD3.40
  Bottom 0.2: v32,48.87 31.16,49.62 20.37,49.62 20.01,49.99 19.02,49.99 18.39,49.35 6.64,49.35 5.9,48.61 v5.9,48.55 | v8.41,24.15 v17.81,15.07
D6  (via drill 0.6 pad 0.7)
  Top 0.2: v43.79,20.46 44.42,21.1 45.27,21.1 IC2.17
  Bottom 0.2: v43.79,20.46 45.06,21.73 45.06,23.95 46.33,25.22 46.33,26.02 45.85,26.49 40.3,26.49 39.66,27.13 37.12,27.13 33.95,23.95 33.95,19.51 30.45,16.01 BOARD3.31
D7
  Top 0.2: IC2.5 43.57,31.82 41.5,31.82 37.44,27.76 37.44,27.13 32.68,22.37 32.68,19.83 29.82,16.97 27.83,16.97 27.77,17.02 27.77,12.62 BOARD3.33
DB4  (via drill 0.6 pad 0.7)
  Top 0.2: v55.7,25.54 53.95,25.54 52.52,26.97 49.19,26.97 49.03,27.13 49.03,28.4 48.55,28.87 47.12,28.87 46.81,28.56 46.81,27.29 47.28,26.81 47.28,23.32 46.65,22.68 45.38,22.68 44.74,23.32 44.74,23.95 43.73,23.95 IC2.15
  Bottom 0.2: v55.7,25.54 55.7,25.38 57.12,23.95 57.12,23.32 59.03,21.41 59.03,16.49 61.09,14.43 62.52,14.43 63.47,13.47 BOARD3.5
DB5  (via drill 0.6 pad 0.7)
  Top 0.2: v60.97,34.62 60.97,35.02 59.37,35.02 IC2.48
  Bottom 0.2: v60.97,34.62 62.77,32.82 62.77,32.02 63.57,31.22 63.57,25.85 65.77,23.62 66.84,22.56 66.81,22.52 66.81,21.89 67.6,21.1 69.35,21.1 69.82,20.62 69.82,19.03 70.3,18.56 73,18.56 73.32,18.24 73.32,12.05 72.49,11.22 67.97,11.22 67.37,10.62 67.37,9.28 65.7,7.6 63.2,7.6 60.97,9.82 BOARD3.8
DB6  (via drill 0.6 pad 0.7)
  Top 0.2: v72.26,9.58 69.46,9.11 67.77,7.42 67.74,7.42 66.97,6.65 62.95,6.65 62.17,7.42 62.17,10.74 60.97,11.94 60.97,12.42 BOARD3.7 | v39.77,33.42 43.57,33.42 IC2.3 | v29.82,38.56 32.68,38.56 34.9,40.78 37.6,40.78 38.39,39.99 45.54,39.99 46.33,40.78 56.62,40.78 v58.77,38.62
  Bottom 0.2: v58.77,38.62 58.97,38.42 65.77,38.42 67.86,36.34 72.05,36.34 74.9,33.48 74.9,31.26 | v72.26,9.58 73.42,9.63 74.27,10.48 74.27,30.46 74.84,31.17 | v39.77,33.42 39.72,33.42 39.72,34.69 39.03,35.38 37.76,35.38 35.22,37.92 30.45,37.92 v29.82,38.56 28.55,37.6 18.55,37.6 16.01,40.14 15.53,40.14 JP2.2 | 74.85,31.2 74.9,31.26 | 74.84,31.17 74.9,31.26 | JP1.13 68.55,30.78 69.03,31.26 74.73,31.26 | 74.73,31.26 74.83,31.16 | 74.73,31.26 74.77,31.22 74.84,31.17
DB7  (via drill 0.6 pad 0.7)
  Top 0.2: v38.92,25.68 41.77,28.62 43.57,28.62 IC2.9
  Bottom 0.2: BOARD3.2 68.57,9.82 66.17,7.42 66.15,7.42 65.54,6.81 61.89,6.81 61.41,7.28 39.51,7.28 39.37,7.42 39.37,10.42 40.17,11.22 40.97,11.22 41.57,11.82 41.97,11.82 41.97,25.45 41.88,25.54 39.06,25.54 v38.92,25.68
E  (via drill 0.6 pad 0.7)
  Top 0.2: IC2.8 47.83,29.43 v47.92,29.67 | v77.29,13.16 70.62,13.16 70.14,13.63 66.81,13.63 66.17,13 66.17,12.68 BOARD3.3
  Bottom 0.2: v47.92,29.67 47.6,29.35 45.69,31.26 45.69,33.16 40.93,37.92 40.3,37.92 36.49,41.73 36.49,44.43 36.8,44.75 36.8,48.56 38.23,49.83 65.06,49.83 66.49,48.56 74.43,48.56 77.29,45.7 v77.29,13.16
ENABLE  (via drill 0.6 pad 0.7)
  Top 0.2: v55.97,14.22 55.97,19.62 54.97,20.62 54.97,21.22 IC2.29
  Bottom 0.2: v55.97,14.22 57.17,13.02 57.17,11.62 56.97,11.62 55.97,10.62 55.97,10.02 BOARD3.12
EXT  (via drill 0.6 pad 0.7)
  Top 0.2: IC2.46 59.1,33.32 57.6,33.32 56.81,32.53 56.01,32.53 v55.54,32.05
  Bottom 0.2: v55.54,32.05 55.38,32.37 53.63,30.62 53.63,29.35 53,28.71 53,27.44 53.95,26.49 53.95,16.49 52.68,15.22 52.68,15.06 52.04,14.43 52.04,11.25 BOARD3.14
GND  (via drill 0.6, 0.6 pad 0.7)
  Top 0.2: IC4.2 13.62,33.19 12.82,33.19 12.16,32.53 C1.1 10.93,31.89 IC1.14 | 48.57,11.22 48.5,11.25 | 37.77,8.62 37.77,8.71 | 46.77,15.62 46.67,15.46 | 51.97,9.62 52.04,9.46 | 52.97,11.42 52.97,11.25 | 40.57,8.82 40.57,8.71 | 43.97,14.02 44.13,14.02 | 43.17,11.42 43.17,11.25 | 3.57,24.82 3.57,24.75 | 4.17,24.82 4.17,24.75 | 3.97,24.82 3.97,24.75 | 50.17,14.62 50.22,14.62
  Top 0.406: v26.09,34.22 26.09,34.51 26.96,35.38 IC5.2
  Bottom 0.2: v10.46,24.31 v13.41,24.31
  other vias: 2.51,48.08 67.13,2.68 48.23,38.56 51.09,23 55.22,23.79 56.17,29.03 54.27,27.76 80.78,48.56 79.67,10.46 64.59,22.52 7.59,46.81 2.51,17.6 78.87,22.52 55.54,33.79 36.46,24.59 40.97,15.42 17.87,23.63 15.94,33.42 6.69,25.14 13.47,12.68 9.66,12.36 10.61,18.87 32.99,40.62 74.43,45.07 78.71,41.57 78.4,30.94 44.74,15.06 50.93,17.76 56.81,46.97 25.22,16.81 21.56,13.95 75.7,39.83 80.46,18.4 74.43,36.02 75.7,15.38 73.16,29.98 45.54,18.08 19.02,3.95 46.81,32.52 51.25,32.05 58.24,8.24 52.2,47.13 43.95,41.1 39.34,41.1 31.52,30.46 7.28,19.67
  pour Bottom: -0.03,50.62 83.57,50.62 83.57,-0.18 -0.03,-0.18
  pour Top (isolate 0.305): -0.03,50.62 83.57,50.62 83.57,-0.1 -0.03,-0.1
HELL
  Top 0.2: BOARD3.6 63.57,9.82 63.57,8.02 64,7.6 65.7,7.6 67.37,9.28 67.37,10.62 67.77,11.02 68.09,11.22 68.97,11.22 69.77,10.74 77.29,10.74 82.21,15.65 82.21,43.96 76.49,49.67 R5.S
MPX_C
  Top 0.2: IC6.9 7.59,12.52 10.13,9.98 BOARD3.42
N$1
  Bottom 0.2: 68.55,-0.18 16.48,-0.18 16.48,8.08 -0.03,8.08
N$2
  Top 0.2: R4.1 17.77,45.39 17.77,45.41 IC3.2
N$3
  Bottom 0.2: 83.79,8.08 69.82,8.08 69.82,0.14
N$4
  Top 0.2: IC1.1 2.2,34.43 1.56,33.79 1.56,27.13 1.88,26.81 IC1.7
N$5
  Top 0.2: R3.1 39.31,20.9 36.65,18.24 36.33,18.24 35.22,17.13 35.22,14.27 35.53,13.95 BOARD3.27
N$6
  Top 0.2: Q2.B 62.91,18.08 R1.1 61.38,18.26 61.57,18.08 60.66,19.19 R2.2
N$7  (via drill 0.6)
  Top 0.2: v39.03,15.54 39.03,13.95 39.34,13.63 39.34,11.25 BOARD3.26
  Bottom 0.2: R6.2 40.46,16.97 v39.03,15.54
N$8
  Top 0.2: 69.82,-0.18 69.82,8.08 83.48,8.08
N$10
  Top 0.2: 16.48,8.08 16.48,8.02 | 16.48,8.02 16.48,-0.18 | 0.13,8.08 16.33,8.08 16.37,8.02 16.48,8.02 | 16.57,8.02 16.48,8.02
N$11
  Top 0.2: IC1.15 7.91,33.16 7.28,32.53 7.28,31.89 6.01,30.62 6.01,29.35 7.28,28.08 7.28,26.49 8.23,25.54 IC1.9
N$15
  Top 0.2: IC5.7 26.33,29.03 24.74,30.62 24.74,34.43 26.96,36.65 IC5.1
N$17  (via drill 0.6 pad 0.7)
  Top 0.2: IC4.7 v16.17,26.81 | v17.75,34.11 17.12,34.43 IC4.1 13.63,34.43
  Bottom 0.2: v16.17,26.81 18.71,26.81 19.66,27.76 19.66,33.79 19.34,34.11 v17.75,34.11
N$18
  Top 0.2: IC4.9 20.93,25.54 23.15,27.76 23.15,31.26 21.25,33.16 IC4.15
OSC_OFF
  Top 0.2: IC2.41 59.13,29.35 58.08,29.35 57.44,28.71 57.44,23.32 59.03,21.73 59.03,16.49 61.09,14.43 64.43,14.43 64.74,14.11 64.74,11.25 BOARD3.4
PD9  (via drill 0.6 pad 0.7)
  Top 0.2: 47.92,36.73 IC2.61 47.76,36.78 47.76,35.86 47.6,35.7 47.6,33.79 50.62,30.78 50.62,29.67 50.93,29.35 54.27,29.35 55.22,28.4 v56.01,27.44 | v60.62,21.25 61.89,21.25 62.05,21.1 62.05,20.22 | 62.05,20.22 62.05,20.2 | R1.2 62.02,20.22 62.05,20.22
  Bottom 0.2: 58.24,23.64 58.24,25.22 v56.01,27.44 | 58.24,23.64 | 58.24,23.64 v60.62,21.25
PR1  (via drill 0.6 pad 0.7)
  Top 0.2: IC2.58 50.21,35.95 v51.73,33.79
  Bottom 0.2: v51.73,33.79 53.63,33.79 54.27,34.43 54.27,37.13 55.7,38.56 56.81,38.56 58.39,40.14 58.39,42.82 SW3.C 58.39,42.94 58.39,43.64 59.35,44.59 61.25,44.59 63.16,42.68 JP1.3
PR2  (via drill 0.6, 0.6 pad 0.7)
  Top 0.2: IC2.59 49.41,35.64 50.14,34.91 v50.14,33.16 | v58.71,46.34 59.66,45.38 60.62,45.38 62.36,43.64 62.36,41.89 60.3,39.83 v59.51,39.83
  Bottom 0.2: v50.14,33.16 50.14,34.43 44.9,39.67 43,39.67 39.19,43.48 39.19,46.79 SW1.2 39.24,47.03 40.3,48.08 56.97,48.08 v58.71,46.34 | JP1.7 68.24,37.6 66.01,39.83 v59.51,39.83
PR3  (via drill 0.6, 0.6 pad 0.7)
  Top 0.2: IC2.60 48.61,34.53 v48.71,34.43 | v34.9,43.96 v38.07,43.96 | v63,48.56 76.17,48.56 81.25,43.48 81.25,33.95 v81.1,33.79 | v78.24,33.64 v73,33.64
  Bottom 0.2: v48.71,34.43 48.71,35.06 44.74,39.03 43,39.03 v38.07,43.96 38.07,45.38 37.76,45.7 37.76,47.77 38.71,48.72 62.36,48.72 v63,48.56 | SW2.2 28.96,46.81 32.68,46.81 34.9,44.59 v34.9,43.96 | v81.1,33.79 v78.24,33.64 | v73,33.64 72.21,33.64 72.05,33.79 69.82,33.79 JP1.9
PR4  (via drill 0.6, 0.6 pad 0.7)
  Top 0.2: SW4.2 47.95,46.84 46.33,45.23 44.74,45.23 43.47,46.49 40.93,46.49 39.66,45.23 v35.85,45.23 | v38.23,36.49 41.09,36.49 v41.57,36.02 41.88,35.7 41.88,34.75 42.4,34.23 IC2.2 | JP1.19 68.71,22.37 69.98,21.1 75.54,21.1 79.35,24.9 79.35,38.88 76.81,41.42 v73,41.42
  Bottom 0.2: v38.23,36.49 38.23,36.81 36.65,38.4 32.52,38.4 31.41,39.51 21.72,39.51 17.91,43.32 16.96,43.32 15.53,44.75 7.59,44.75 JP2.8 | v35.85,45.23 35.85,41.42 39.98,37.29 40.3,37.29 v41.57,36.02 | 69.82,41.42 69.82,43.32 69.19,43.96 63,43.96 61.89,45.07 57.28,45.07 56.17,46.18 50.55,46.18 SW4.2 | v73,41.42 69.82,41.42 | 69.82,41.42 JP1.5
RESET  (via drill 0.6)
  Top 0.2: IC2.20 47.81,24.8 v48.23,25.22 | v20.77,42.84 20.61,42.84 19.58,43.88 | 19.58,43.88 19.5,43.96 19.5,44.75 R4.2 20.5,44.91 C3.1 | JP2.9 JP2.10 5.05,43.16 6.32,44.43 15.85,44.43 16.96,43.32 19.02,43.32 19.58,43.88 | v75.38,18.71 75.22,18.56 69.03,18.56 68.55,19.03 JP1.21 | v59.66,41.26 57.92,41.26 57.6,41.42 54.74,41.42 54.11,42.05 29.03,42.05 28.55,41.57 R7.1 | R7.1
  Bottom 0.2: v20.77,42.84 22.04,41.57 R7.1 28.23,41.42 28.23,40.3 28.55,39.99 31.88,39.99 32.52,39.35 36.8,39.35 40.46,35.7 40.46,34.75 42.04,33.16 43,33.16 47.28,28.87 47.28,27.44 47.76,26.97 47.76,25.86 48.23,25.38 v48.23,25.22 | v59.66,41.26 65.38,41.26 67.76,38.88 74.27,38.88 76.33,36.81 76.33,19.67 v75.38,18.71
RS  (via drill 0.6 pad 0.7)
  Top 0.2: IC2.44 59.11,31.73 57.92,31.73 56.33,30.14 v51.57,30.14
  Bottom 0.2: v51.57,30.14 51.57,26.97 52.68,25.86 52.68,22.68 52.2,22.21 52.2,16.65 52.04,16.49 50.14,16.49 47.76,14.11 46.33,14.11 45.69,13.47 BOARD3.19
SCAN  (via drill 0.6 pad 0.7)
  Top 0.2: v54.57,15.22 54.57,20.22 54.17,20.62 54.17,21.22 IC2.28
  Bottom 0.2: v54.57,15.22 54.57,8.02 42.37,8.02 40.57,9.82 BOARD3.24
SP1
  Top 0.2: IC2.40 59.29,28.56 60.46,28.56 62.2,30.3 62.2,39.83 66.33,43.96 70.3,43.96 70.94,44.59 70.94,45.07 JP1.2
SP2
  Top 0.2: IC2.39 59.28,27.76 60.62,27.76 62.84,29.99 62.84,39.19 65.06,41.42 70.46,41.42 71.09,42.05 JP1.4
SP3
  Top 0.2: 59.3,27.13 IC2.38 59.27,26.97 61.09,26.97 63.47,29.35 63.47,38.56 64.11,39.19 67.44,39.19 67.76,38.88 70.3,38.88 71.09,39.67 JP1.6
SP4
  Top 0.2: IC2.37 59.27,26.17 61.57,26.17 66.33,30.94 66.33,35.54 67.13,36.34 70.62,36.34 70.94,36.65 70.94,37.45 JP1.8
SP5
  Top 0.2: IC2.36 59.26,25.38 61.73,25.38 66.97,30.62 66.97,33.16 67.6,33.79 70.46,33.79 70.94,34.27 70.94,34.91 JP1.10
SP6
  Top 0.2: IC2.35 59.25,24.59 62.2,24.59 62.2,25.06 67.44,30.3 67.44,31.1 67.6,31.26 70.62,31.26 71.09,31.73 JP1.12
SP7  (via drill 0.6 pad 0.7)
  Top 0.2: v61.09,23.16 63.32,23.16 63.32,25.22 66.81,28.71 70.78,28.71 71.09,29.03 JP1.14 | IC2.42 59.66,30.3 60.3,30.3 v61.09,31.1
  Bottom 0.2: v61.09,23.16 v61.09,31.1
SWEEPHOLD
  Top 0.2: JP1.16 71.09,26.65 70.62,26.17 67.44,26.17 65.86,24.59 65.86,21.57 Q2.C
TCK  (via drill 0.6 pad 0.7)
  Top 0.2: IC2.57 51.01,37.69 v49.82,38.56 | JP2.7 7.59,38.24 10.13,35.7 20.29,35.7 26.01,41.42 26.33,41.42 26.33,41.73 27.6,43 28.55,43 29.18,42.53 45.06,42.53 46.49,43.8 v47.6,43.8
  Bottom 0.2: v47.6,43.8 47.6,41.42 49.82,39.19 v49.82,38.56
TDI  (via drill 0.6 pad 0.7)
  Top 0.2: IC2.54 53.31,36.93 53.31,37.92 v53.95,38.56 | JP2.1 20.29,37.92 27.28,45.23 29.5,45.23 31.09,46.81 32.36,46.81 33.95,48.4 53,48.4 53.95,47.45 v53.95,44.11
  Bottom 0.2: v53.95,44.11 v53.95,38.56
TDO  (via drill 0.6 pad 0.7)
  Top 0.2: JP2.5 11.4,39.19 19.98,39.19 26.01,45.23 26.01,47.77 26.96,48.72 30.45,48.72 31.41,47.77 32.36,47.77 33.63,49.03 53.95,49.03 55.22,48.08 v55.22,45.23 | v52.68,35.06 52.68,36.76 IC2.55
  Bottom 0.2: v52.68,35.06 52.68,38.56 53,38.88 53,45.23 v55.22,45.23
TIME_A  (via drill 0.6 pad 0.7)
  Top 0.2: v59.67,5.66 59.67,6.82 59.68,6.82 59.66,6.97 59.66,12.93 57.57,15.02 57.57,21.22 IC2.32 | v22.17,6.42 18.97,9.62 18.97,10.42 18.17,11.22 10.77,11.22 10.77,14.46 10.21,14.71 10.21,16.07 IC6.11
  Bottom 0.2: v59.67,5.66 22.93,5.66 v22.17,6.42
TIME_B  (via drill 0.6 pad 0.7)
  Top 0.2: 31.63,8.02 31.72,8.02 | 31.72,8.02 53.17,8.02 54.57,9.42 54.57,10.62 54.97,11.02 54.97,11.22 56.37,11.22 57.17,12.02 57.17,14.02 56.97,14.22 56.97,20.22 56.57,20.62 56.57,21.22 IC2.31 | v9.21,14.07 8.81,14.47 8.81,16.07 IC6.10 | 31.72,8.02 31.72,10.62 31.09,11.25 29.5,11.25 29.18,11.57 29.18,15.64 v29.08,15.74
  Bottom 0.2: v29.08,15.74 29,15.02 28.96,15.06 20.29,15.06 19.3,14.07 v9.21,14.07
TMS  (via drill 0.6 pad 0.7)
  Top 0.2: IC2.56 51.81,38.16 v51.41,38.56 | JP2.3 12.67,37.6 13.63,36.34 19.98,36.34 27.6,43.96 28.87,43.96 29.82,43 44.74,43 46.49,44.75 48.71,44.75 v49.35,44.11
  Bottom 0.2: v49.35,44.11 49.35,40.62 v51.41,38.56
TRIGGER
  Top 0.2: 51.73,21.15 IC2.25 51.89,21.16 51.89,20.3 52.04,20.14 52.04,15.38 50.77,14.11 BOARD3.15

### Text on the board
tNames: 41 | 39 | 37 | 35 | 33 | 31 | 29 | 27 | 25 | 23 | 21 | 19 | 17 | 15 | 13 | 11 | 9 | 7 | 5 | 3 | 1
